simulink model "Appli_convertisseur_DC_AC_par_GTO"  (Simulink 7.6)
settings: Solver=ode23tb  StartTime=0.0  StopTime=T  RelTol=1e-3
InitFcn:
  | T=1/60;
StopFcn:
  | close all
  | load Igen_Ualim.mat
  | subplot 211
  | plot(x(1,:),x(2,:))
  | grid
  | axis([0 0.018 -11 11])
  | title('tension d''alimentation')
  | xlabel('temps')
  | 
  | subplot 212
  | plot(x(1,:),x(3,:))
  | axis([0 0.018 0.05 0.35])
  | title('Courant fourni par le générateur')
  | grid
  | xlabel('temps')
libraries: powerlib x10, powerlib_extras x1

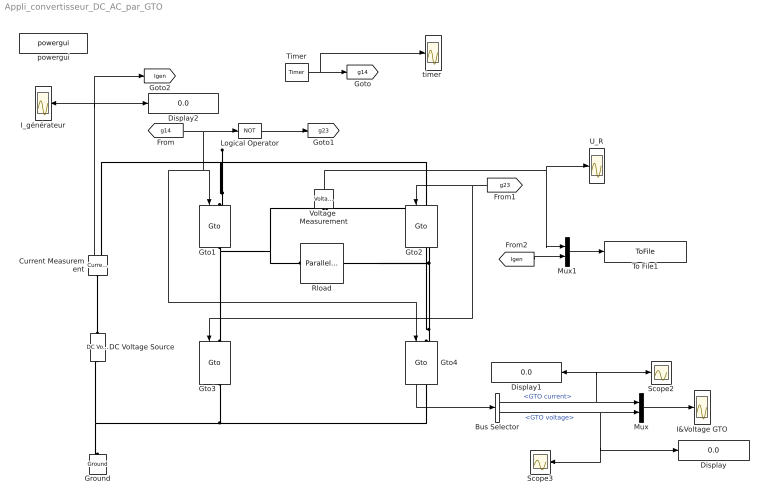
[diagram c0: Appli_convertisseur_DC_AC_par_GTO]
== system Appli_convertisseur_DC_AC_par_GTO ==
  Bus Selector : BusSelector  OutputSignals=GTO current,GTO voltage
  Current Measurement : powerlib/Measurements/Current Measurement  DialogController=POWERSYS.PowerSysDialog  SystemSampleTime=-1  PhasorSimulation=off  OutputType=Complex  PSBequivalent=0
  DC Voltage Source : powerlib/Electrical Sources/DC Voltage Source  DialogController=POWERSYS.PowerSysDialog  SystemSampleTime=-1  Amplitude=12  Measurements=None
  Display : Display
  Display1 : Display
  Display2 : Display
  Ground : powerlib/Elements/Ground  DialogController=POWERSYS.PowerSysDialog  PhysicalDomain=powersysdomain  SubClassName=unknown  LeftPortType=p1  RightPortType=p1  LConnTagsString=a
  Gto{1..4} (4 alike) : powerlib/Power Electronics/Gto  DialogController=POWERSYS.PowerSysDialog  SystemSampleTime=-1  Ron=0.001  Lon=0  Vf=1  Tf=10e-6  Tt=20e-6  IC=0  Rs=1e5  Cs=inf  Measurements=on
  I&Voltage GTO : Scope
  I_générateur : Scope
  Logical Operator : Logic  Operator=NOT  AllPortsSameDT=off  OutDataTypeStr=boolean
  Mux : Mux  Inputs=2
  Mux1 : Mux  Inputs=2
  Rload : powerlib/Elements/Parallel RLC Branch  DialogController=POWERSYS.PowerSysDialog  PhysicalDomain=powersysdomain  SubClassName=unknown  LeftPortType=p1  RightPortType=p1  LConnTagsString=a  RConnTagsString=__new0  BranchType=R  Resistance=100  Inductance=1e-3  SetiL0=off  InitialCurrent=0  Capacitance=1e-6  Setx0=off  InitialVoltage=0  Measurements=None
  Scope2 : Scope
  Scope3 : Scope
  Timer : powerlib_extras/Control  Blocks/Timer  DialogController=POWERSYS.PowerSysDialog  SystemSampleTime=-1  t="[0 0.19  0.2 0.4 0.401 0.59 0.6 0.8 0.81 1]*T"  e="[0 0 1 1  0 0 1 1 0 0]"
  To File1 : ToFile  Filename=Igen_Ualim  MatrixName=x
  U_R : Scope
  Voltage  Measurement : powerlib/Measurements/Voltage Measurement  DialogController=POWERSYS.PowerSysDialog  SystemSampleTime=-1  PhasorSimulation=off  OutputType=Complex  PSBequivalent=0
  powergui : powerlib/powergui  Priority=2  SystemSampleTime=-1  SimulationMode=Continuous  SampleTime=0  frequency=60  SPID=off  DisableSnubberDevices=off  DisableRonSwitches=off  DisableVfSwitches=off  SwTol=0  Interpol=off  frequencyindice=0  echomessages=off  HookPort=off  DisplayEquations=off  FunctionMessages=off  EnableUseOfTLC=off  x0status=blocks  RestoreLinks=warning  ResistiveCurrentMeasurement=off  Frange=logspace(0,3,50)  Ylog=off  Xlog=off  ShowGrid=off  save=off  variable=ZData  ZoomFFT=on  StartTime=0.0  cycles=1  DisplayStyle=off  fundamental=60  FreqAxis=off  MaxFrequency=1000  frequencyindicesteady=1  RmsSteady=1  display=off  Ts=0  methode=off
  "timer " : Scope
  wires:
  Voltage  Measurement/1 -> U_R/1, Mux1/1
  [g14] -> Gto4/1, Gto1/1, Logical Operator/1
  [g23] -> Gto2/1, Gto3/1
  Logical Operator/1 -> [g23]
  Timer/1 -> [g14], "timer "/1
  Gto4/1 -> Bus Selector/1
  Bus Selector/1 -> Mux/1, Display1/1, Scope2/1  "<GTO current>"
  Bus Selector/2 -> Mux/2, Display/1, Scope3/1  "<GTO voltage>"
  Mux/1 -> I&Voltage GTO/1
  Current Measurement/1 -> Display2/1, I_générateur/1, [Igen]
  [Igen] -> Mux1/2
  Mux1/1 -> To File1/1
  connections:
  Gto3/RConn1 -- Ground/LConn1 -- DC Voltage Source/LConn1 -- Gto4/RConn1
  Gto4/LConn1 -- Rload/RConn1 -- Voltage  Measurement/LConn2 -- Gto2/RConn1
  Gto1/RConn1 -- Rload/LConn1 -- Voltage  Measurement/LConn1 -- Gto3/LConn1
  Gto1/LConn1 -- Current Measurement/RConn1 -- Gto2/LConn1
  Current Measurement/LConn1 -- DC Voltage Source/RConn1
